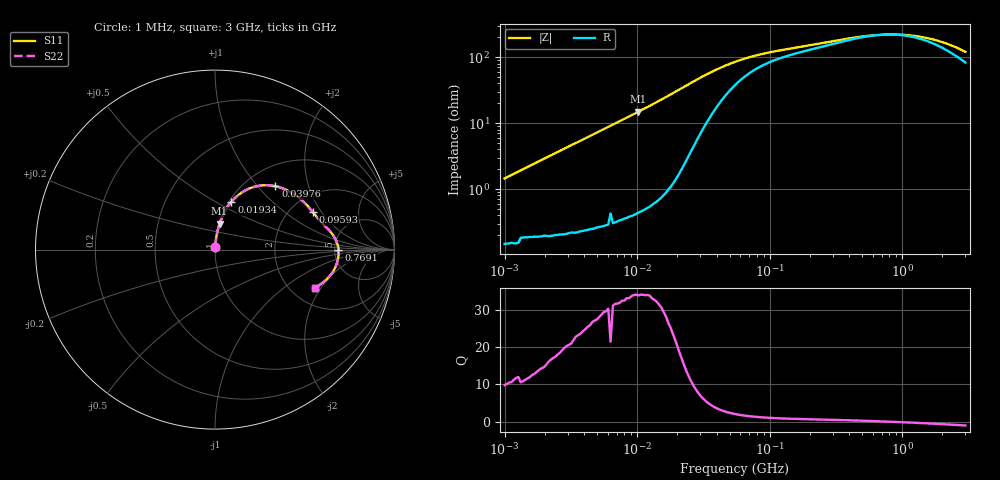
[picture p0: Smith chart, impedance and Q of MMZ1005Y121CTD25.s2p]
! S-Parameter Data Generated by TDK Corporation
! Copyright(C) 2025 TDK Corporation.
! All Rights Reserved.
! TDK P/N: MMZ1005Y121CTD25 (Chip Bead)
! Property: |Z|=120ohm at 100MHz
! Size(LxWxT): 1x0.5x0.5mm
! Model Type: s2p (Touchstone File Format Version 1.0)
! Frequency: DC=Yes Start=1MHz Stop=3000MHz 202points Log-sweep
! Model Generated on Feb. 6, 2025
! Terms and conditions regarding TDK Simulation Models:
! 1)This simulation model is being provided solely for informational
!  purposes. Please refer to the specifications of the products in
!  terms of detailed characteristics of such products.
! 2)In no event shall TDK Corporation of any of its subsidiaries be
!  liable for any loss or damage arising, directly or indirectly,
!  from any information contained in this simulation model, including,
!  but not limited to loss or damages arising from any inaccuracies,
!  omissions or errors in connection with such information.
! 3)Any and all copyrights on this simulation model are owned by
!  TDK Corporation.  Duplication or redistribution of this simulation
!  model without prior written permission from TDK Corporation
!  is prohibited.
! 4)This simulation model is subject to any modification or change
!  without any prior notice.
! 5)Neither TDK Corporation nor any of its subsidiaries shall make any
!  warranty, express or implied, including but not limited to the
!  correctness, implied warranties of merchantability and fitness for
!  a particular purpose with respect to this simulation models.
! 6)The use of this simulation model shall be deemed to have consented
!  to the terms and conditions hereof.
! Port Assignments:
!  1 ---@@@--- 2
! Applicable Conditions:
!  Temperature = 25 degC
!  DC Bias Current = 0 A
!  Small Signal Operation
# Hz S MA R 50
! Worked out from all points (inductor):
!   201 points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, 1 MHz to 3 GHz, reference 50 ohm
!   read as one part in series: L = 230 nH near 1.041 MHz
!   highest Q = 34.1 at 10.19 MHz (marker M1), where L = 232 nH
!   self-resonance near 757.9 MHz
!   S11 on the Smith chart (normalised r, x): 1 MHz: 1.00, +0.03; 19.34 MHz: 1.03, +0.59; 39.76 MHz: 1.35, +1.25; 95.93 MHz: 2.62, +1.67; 769.1 MHz: 5.41, -0.04; 3 GHz: 2.66, -1.74
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1000000  0.01446 83.3  0.9984 -0.8  0.9984 -0.8  0.01446 83.3
3900413  0.05613 84.4  0.9961 -3.2  0.9961 -3.2  0.05613 84.4
6563319  0.09414 82.8  0.9925 -5.4  0.9925 -5.4  0.09414 82.8
1.019448e7  0.1463 79.9  0.9849 -8.4  0.9849 -8.4  0.1463 79.9
1.461624e7  0.2108 76.0  0.9708 -12.2  0.9708 -12.2  0.2108 76.0
1.934349e7  0.2812 71.1  0.947 -16.3  0.947 -16.3  0.2812 71.1
2.362996e7  0.3418 65.8  0.9147 -19.9  0.9147 -19.9  0.3418 65.8
2.886629e7  0.4047 59.0  0.864 -23.7  0.864 -23.7  0.4047 59.0
3.387922e7  0.4502 52.8  0.811 -26.2  0.811 -26.2  0.4502 52.8
3.976269e7  0.488 46.4  0.7515 -28.0  0.7515 -28.0  0.488 46.4
5.477226e7  0.5395 34.7  0.6357 -28.9  0.6357 -28.9  0.5395 34.7
6.964249e7  0.5627 27.8  0.5666 -27.6  0.5666 -27.6  0.5627 27.8
9.593103e7  0.5836 21.1  0.5018 -24.8  0.5018 -24.8  0.5836 21.1
1.321429e8  0.6006 16.5  0.4574 -21.9  0.4574 -21.9  0.6006 16.5
2.136344e8  0.6284 11.8  0.406 -18.5  0.406 -18.5  0.6284 11.8
4.951867e8  0.6767 4.3  0.3291 -8.9  0.3291 -8.9  0.6767 4.3
7.691493e8  0.6881 -0.2  0.3119 0.4  0.3119 0.4  0.6881 -0.2
8.005644e8  0.6885 -0.6  0.3117 1.3  0.3117 1.3  0.6885 -0.6
1.10276e9  0.6873 -4.3  0.3186 9.2  0.3186 9.2  0.6873 -4.3
1.519029e9  0.677 -8.5  0.345 16.8  0.345 16.8  0.677 -8.5
2.177892e9  0.6479 -14.3  0.4052 23.3  0.4052 23.3  0.6479 -14.3
3e9  0.594 -20.9  0.493 25.5  0.493 25.5  0.594 -20.9
